(* Logix 5000 DataType export Yaskawa_AOI_Status_Bits; software revision 17.00 *)

TYPE Yaskawa_AOI_Status_Bits :   // Internal bits used to interlock Yaskawa AOI execution. v2.4.0
STRUCT
   MAM : BOOL;   // Move AOI Active
   MAJ : BOOL;   // Jog AOI Active
   MAB : BOOL;   // Blending AOI Active
   MAG : BOOL;   // Gearing AOI Active
   MAHSP : BOOL;   // Home SetPoint AOI Active
   MAH : BOOL;   // Homing AOI Active
   MSQE : BOOL;   // Sequence Edit AOI Active
   MSQR : BOOL;   // Sequence Run AOI Active
   MHSI : BOOL;   // High Speed Index AOI Active
   MSO : BOOL;   // Servo On
   MSF : BOOL;   // Servo Off
   MAFR : BOOL;   // Fault Reset
   MAS : BOOL;   // Servo Abort
   MTRQ : BOOL;   // Torque Mode Active
   MPLS : BOOL;   // PLS Active
   MCLK : BOOL;   // SetClock Active
   MSTL : BOOL;   // Set Torque Limit Active
   AOI_Permissive : BOOL;   // Permissive to Execute an AOI
END_STRUCT
END_TYPE
